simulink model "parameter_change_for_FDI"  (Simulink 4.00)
settings: Solver=ode45  StartTime=0.0  StopTime=1020  RelTol=1e-3

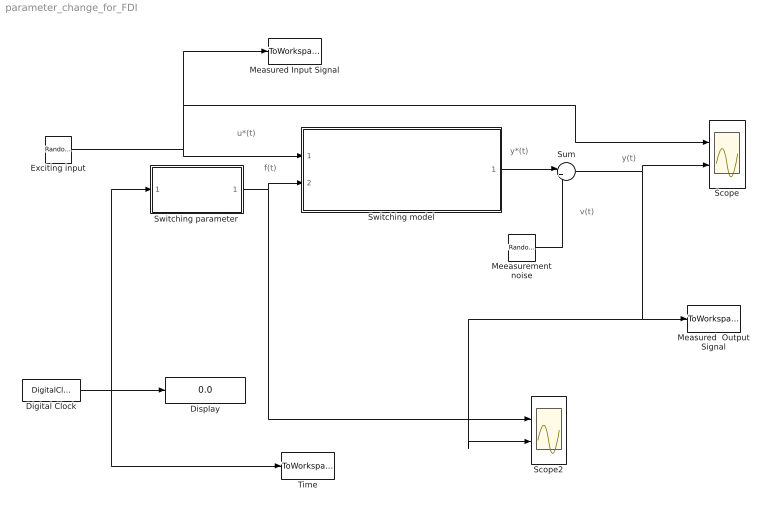
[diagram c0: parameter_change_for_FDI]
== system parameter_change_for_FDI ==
  note: u*(t)
  note: y(t)
  note: y*(t)
  note: v(t)
  note: f(t)
  " Measured Input Signal " : ToWorkspace  VariableName=U  SampleTime=1  SaveFormat=Array
  Digital Clock : DigitalClock  SampleTime=1
  Display : Display
  Exciting input : RandomNumber  Mean=0  Variance=0.4/(0.6388)^2  Seed=1  SampleTime=1
  Measured  Output Signal : ToWorkspace  VariableName=Y  SampleTime=1  SaveFormat=Array
  Meeasurement noise : RandomNumber  Mean=0  Variance=(0.01)^2  Seed=3  SampleTime=1
  Scope : Scope  NumInputPorts=2
  Scope2 : Scope  NumInputPorts=2
  Sum : Sum  Inputs=|++  SaturateOnIntegerOverflow=on
  Switching parameter : Subsystem
  Switching model : Subsystem
  Time : ToWorkspace  VariableName=t  SampleTime=1  SaveFormat=Array
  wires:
  Exciting input/1 -> Switching model/1(u*(t)), " Measured Input Signal "/1, Scope/1
  Digital Clock/1 -> Display/1, Time/1, Switching parameter/1(t)
  Switching parameter/1(a(t)) -> Switching model/2(f(t)), Scope2/1
  Meeasurement noise/1 -> Sum/2
  Switching model/1(y*(t)) -> Sum/1
  Sum/1 -> Scope/2, Scope2/2, Measured  Output Signal/1

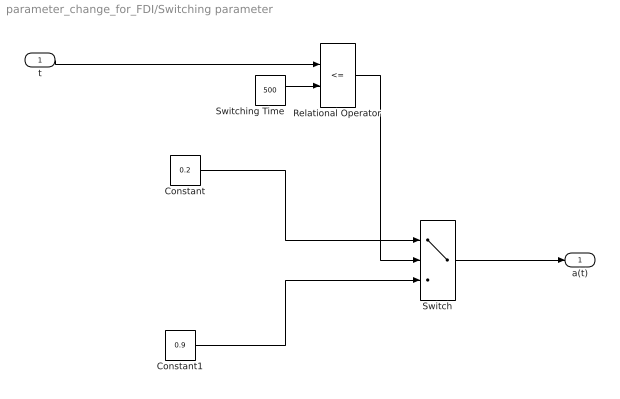
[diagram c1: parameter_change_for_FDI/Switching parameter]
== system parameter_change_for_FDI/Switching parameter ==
  t : Inport  Port=1  LatchInput=off
  Constant : Constant  Value=0.2
  Constant1 : Constant  Value=0.9
  Relational Operator : RelationalOperator  Operator=<=
  Switch : Switch  Threshold=1
  Switching Time : Constant  Value=500
  a(t) : Outport  Port=1
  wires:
  Constant/1 -> Switch/1
  Constant1/1 -> Switch/3
  Switching Time/1 -> Relational Operator/2
  Relational Operator/1 -> Switch/2
  Switch/1 -> a(t)/1
  t/1 -> Relational Operator/1

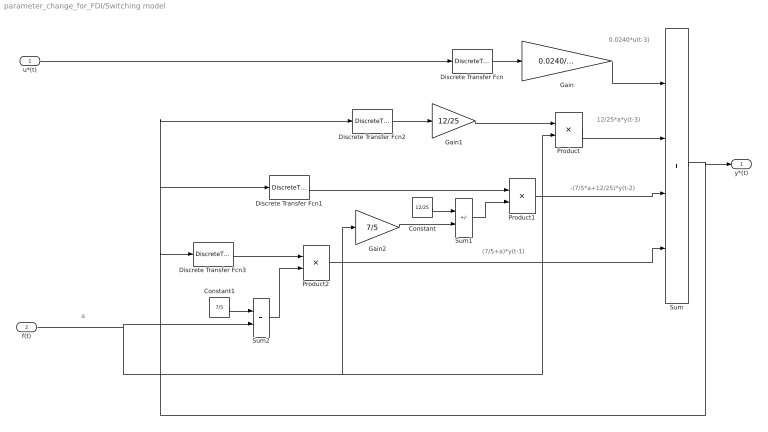
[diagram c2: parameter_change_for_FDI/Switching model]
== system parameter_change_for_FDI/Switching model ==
  note: 0.0240*u(t-3)
  note: 12/25*a*y(t-3)
  note: -(7/5*a+12/25)*y(t-2)
  note: a
  note: (7/5+a)*y(t-1)
  u*(t) : Inport  Port=1  LatchInput=off
  f(t) : Inport  Port=2  LatchInput=off
  Constant : Constant  Value=12/25
  Constant1 : Constant  Value=7/5
  Discrete Transfer Fcn : DiscreteTransferFcn  Numerator=[1]  Denominator=[1 0 0 0]  SampleTime=1  Realization=auto
  Discrete Transfer Fcn1 : DiscreteTransferFcn  Numerator=[1]  Denominator=[1 0 0]  SampleTime=1  Realization=auto
  Discrete Transfer Fcn2 : DiscreteTransferFcn  Numerator=[1]  Denominator=[1 0 0 0]  SampleTime=1  Realization=auto
  Discrete Transfer Fcn3 : DiscreteTransferFcn  Numerator=[1]  Denominator=[1 0]  SampleTime=1  Realization=auto
  Gain : Gain  Gain=0.0240/0.1304  Multiplication=Element-wise(K.*u)  SaturateOnIntegerOverflow=on
  Gain1 : Gain  Gain=12/25  Multiplication=Element-wise(K.*u)  SaturateOnIntegerOverflow=on
  Gain2 : Gain  Gain=7/5  Multiplication=Element-wise(K.*u)  SaturateOnIntegerOverflow=on
  Product : Product  Inputs=2  Multiplication=Element-wise(.*)  SaturateOnIntegerOverflow=on
  Product1 : Product  Inputs=2  Multiplication=Element-wise(.*)  SaturateOnIntegerOverflow=on
  Product2 : Product  Inputs=2  Multiplication=Element-wise(.*)  SaturateOnIntegerOverflow=on
  Sum : Sum  Inputs=++++  SaturateOnIntegerOverflow=on
  Sum1 : Sum  Inputs=--  SaturateOnIntegerOverflow=on
  Sum2 : Sum  Inputs=++  SaturateOnIntegerOverflow=on
  y*(t) : Outport  Port=1
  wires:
  Discrete Transfer Fcn/1 -> Gain/1
  Sum/1 -> y*(t)/1, Discrete Transfer Fcn2/1, Discrete Transfer Fcn1/1, Discrete Transfer Fcn3/1
  Gain/1 -> Sum/1
  u*(t)/1 -> Discrete Transfer Fcn/1
  Discrete Transfer Fcn2/1 -> Gain1/1
  Product/1 -> Sum/2
  Gain1/1 -> Product/1
  Product1/1 -> Sum/3
  Discrete Transfer Fcn1/1 -> Product1/1
  Gain2/1 -> Sum1/2
  Sum1/1 -> Product1/2
  Constant/1 -> Sum1/1
  f(t)/1 -> Sum2/2, Gain2/1, Product/2
  Product2/1 -> Sum/4
  Discrete Transfer Fcn3/1 -> Product2/1
  Constant1/1 -> Sum2/1
  Sum2/1 -> Product2/2
